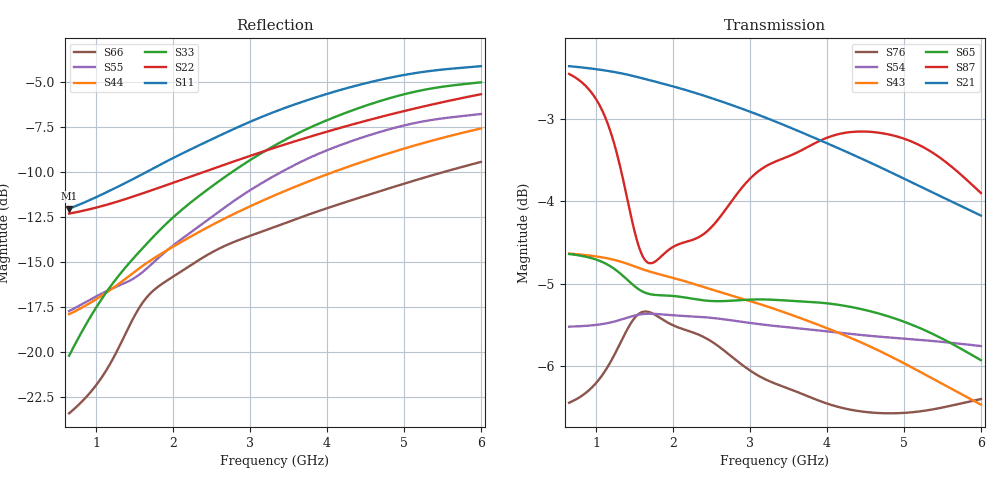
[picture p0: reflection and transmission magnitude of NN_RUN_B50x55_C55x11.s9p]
! IGNION VIRTUAL ANTENNA LIBRARY
! NN_RUN_B50x55_C55x11
! Virtual Antenna™ RUN mXTEND™: NN02-224 12.0 mm x 3.0 mm x 2.4 mm
! https://ignion.io/product/run-mxtend/
! Board: 50 mm x 55 mm
! Clearance Area: 55 mm x 11 mm
! Feeding line: L-shape; 11mm x 2mm and 5mm x 2mm
! Applications: Fleet management, IoT
! Frequency range 0.65GHz to 6GHz, step 10MHz
! Number of ports 9
! This product and its use is protected by at least one or more of the following patents and patent
! applications US 8,203,492 B2; US 8,237,615 B2; PCT/EP2013/064692; WO 2014/012842 A1; US 2019/190122 A1;
! US 62/072,671; and other domestic and international patents pending. Additional information about
! patents related to this product is available at https://ignion.io/files/Patent-list-NN.pdf, all
! rights reserved. Copyright, Ignion 2021.
! Need more help? Your platform is much different than these examples in the manual? Use our
! Fast Track service (https://ignion.io/fast-track/), for free, and get a personalized antenna design in
! just 24 hours.
! Touchstone port 1 = "Series Port"
! Touchstone port 2 = "Shunt Port"
! Touchstone port 3 = "Series Port"
! Touchstone port 4 = "Shunt Port"
! Touchstone port 5 = "Series Port"
! Touchstone port 6 = "Shunt Port"
! Touchstone port 7 = "Series Port"
! Touchstone port 8 = "Shunt Port"
! Touchstone port 9 = "Series Port"
! IE3D S-Parameters Output Version 2.0
# GHZ S MA R 50
! Nport = 9
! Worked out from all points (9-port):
!   536 points, 650 MHz to 6 GHz, reference 50 ohm
!   strongest paths, dB at 650 MHz, 1.99 GHz, 3.33 GHz, 4.67 GHz, 6 GHz:
!     S21: -2.4, -2.6, -3.0, -3.6, -4.2
!     S87: -2.5, -4.6, -3.5, -3.2, -3.9
!     S65: -4.6, -5.1, -5.2, -5.4, -5.9
!     S43: -4.6, -4.9, -5.3, -5.8, -6.5
!     S54: -5.5, -5.4, -5.5, -5.6, -5.8
!     S76: -6.4, -5.5, -6.2, -6.6, -6.4
!   lowest |S11| = -12.0 dB at 650 MHz (marker M1), VSWR 1.67, Z = 31.1 + j7.69 ohm
!   |S11| at or under -10 dB: start of sweep to 1.663 GHz
